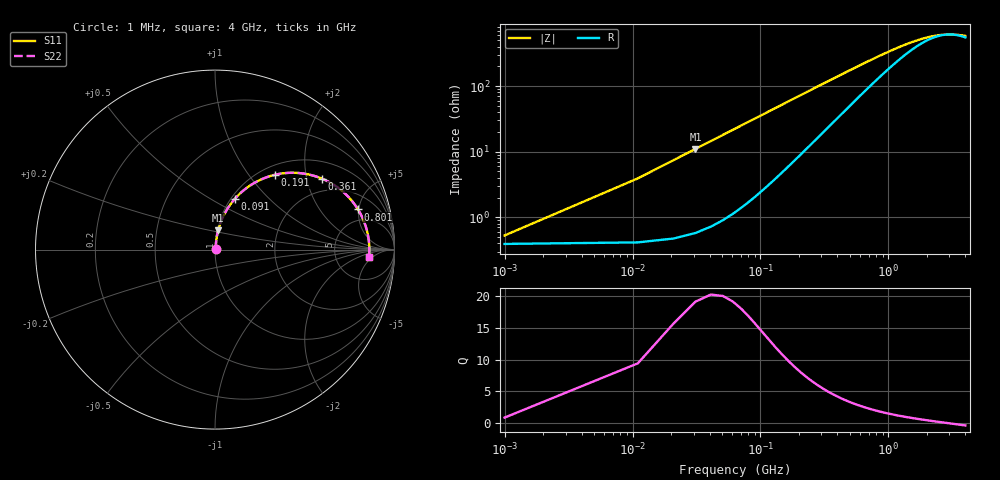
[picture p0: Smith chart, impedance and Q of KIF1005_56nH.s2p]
!version-2
!date-12.2020
!Series
# MHz S RI R 50
!Freq ReS11 ImS11 ReS21 ImS21 ReS12 ImS12 ReS22 ImS22
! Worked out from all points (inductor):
!   401 points, 1 MHz to 4 GHz, reference 50 ohm
!   read as one part in series: L = 56.3 nH near 21 MHz
!   highest Q = 17.9 at 31 MHz (marker M1), where L = 56.3 nH
!   self-resonance near 3.013 GHz
!   S11 on the Smith chart (normalised r, x): 1 MHz: 1.01, +0.01; 91 MHz: 1.04, +0.64; 191 MHz: 1.16, +1.34; 361 MHz: 1.53, +2.49; 801 MHz: 3.45, +4.90; 4 GHz: 12, -4
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1  0.00391 0.00351  0.9961 -0.00351  0.9961 -0.00351  0.00391 0.00351
11  0.00561 0.0385  0.9944 -0.0385  0.9944 -0.0385  0.00561 0.0385
21  0.0101 0.0732  0.9899 -0.0732  0.9899 -0.0732  0.0101 0.0732
31  0.0174 0.1072  0.9826 -0.1072  0.9826 -0.1072  0.0174 0.1072
41  0.0273 0.1402  0.9727 -0.1402  0.9727 -0.1402  0.0273 0.1402
51  0.0397 0.1719  0.9603 -0.1719  0.9603 -0.1719  0.0397 0.1719
71  0.0709 0.2303  0.9291 -0.2303  0.9291 -0.2303  0.0709 0.2303
91  0.1089 0.2811  0.8911 -0.2811  0.8911 -0.2811  0.1089 0.2811
131  0.1966 0.3578  0.8034 -0.3578  0.8034 -0.3578  0.1966 0.3578
191  0.3318 0.4163  0.6682 -0.4163  0.6682 -0.4163  0.3318 0.4163
271  0.4812 0.4253  0.5188 -0.4253  0.5188 -0.4253  0.4812 0.4253
361  0.5978 0.3946  0.4022 -0.3946  0.4022 -0.3946  0.5978 0.3946
491  0.6983 0.335  0.3017 -0.335  0.3017 -0.335  0.6983 0.335
671  0.769 0.2637  0.231 -0.2637  0.231 -0.2637  0.769 0.2637
801  0.7967 0.2238  0.2033 -0.2238  0.2033 -0.2238  0.7967 0.2238
1051  0.8259 0.1672  0.1741 -0.1672  0.1741 -0.1672  0.8259 0.1672
1341  0.8422 0.122  0.1578 -0.122  0.1578 -0.122  0.8422 0.122
1651  0.8509 0.0873  0.1491 -0.0873  0.1491 -0.0873  0.8509 0.0873
2001  0.856 0.0579  0.144 -0.0579  0.144 -0.0579  0.856 0.0579
2671  0.8596 0.0167  0.1404 -0.0167  0.1404 -0.0167  0.8596 0.0167
3341  0.8597 -0.0143  0.1403 0.0143  0.1403 0.0143  0.8597 -0.0143
4000  0.8581 -0.0397  0.1419 0.0397  0.1419 0.0397  0.8581 -0.0397
